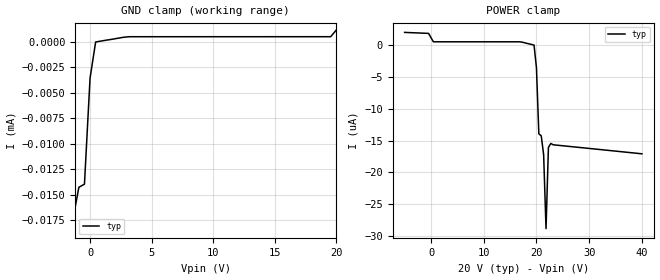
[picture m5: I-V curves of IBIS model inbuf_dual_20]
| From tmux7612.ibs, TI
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| inbuf_dual_20
[Model]   inbuf_dual_20
Model_type   Input
Vinl = 0.8
Vinh = 1.3
|   typ   min   max
C_comp   2.533030e-12   NA   NA
[Voltage Range]   20   NA   NA
[Temperature Range]   27   NA   NA
[Power Clamp Reference]   20   NA   NA
[GND Clamp Reference]   0   NA   NA
[GND Clamp]
|   Voltage   I(typ)   I(min)   I(max)
-25V      -3.924A    NA         NA
-20.91V   -9.933mA   NA         NA
-20.45V   -17.12uA   NA         NA
-2.727V   -15.46uA   NA         NA
-2.273V   -16.07uA   NA         NA
-1.818V   -28.83uA   NA         NA
-1.364V   -17.22uA   NA         NA
-909.1mV  -14.25uA   NA         NA
-454.5mV  -13.95uA   NA         NA
0V        -3.562uA   NA         NA
454.5mV   -16.46nA   NA         NA
20V       1.144uA    NA         NA
[POWER Clamp]
|   Voltage   I(typ)   I(min)   I(max)
-5V       1.977uA    NA         NA
-454.5mV  1.821uA    NA         NA
454.5mV   501.2nA    NA         NA
19.55V    -16.46nA   NA         NA
20V       -3.562uA   NA         NA
20.45V    -13.95uA   NA         NA
20.91V    -14.25uA   NA         NA
21.36V    -17.22uA   NA         NA
21.82V    -28.83uA   NA         NA
22.27V    -16.07uA   NA         NA
22.73V    -15.46uA   NA         NA
40V       -17.08uA   NA         NA
